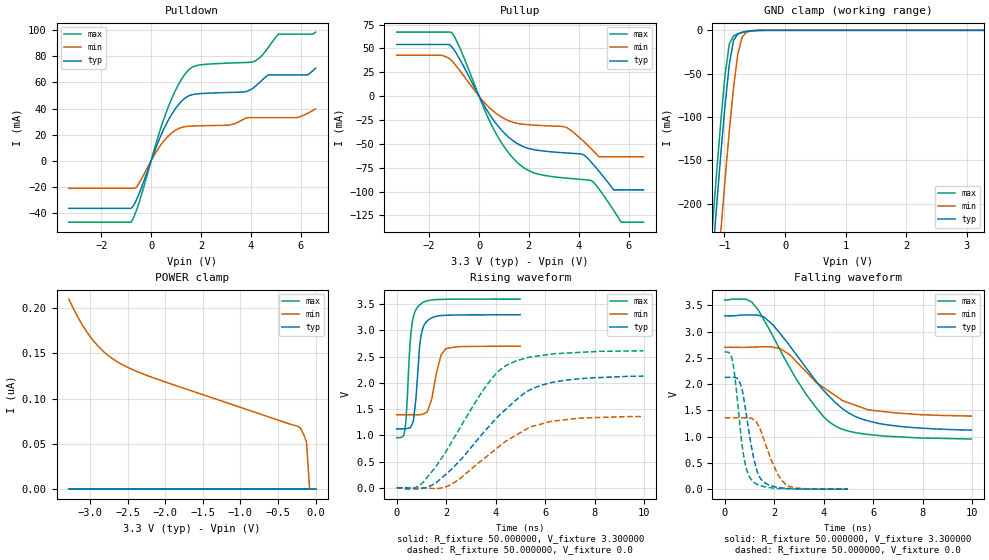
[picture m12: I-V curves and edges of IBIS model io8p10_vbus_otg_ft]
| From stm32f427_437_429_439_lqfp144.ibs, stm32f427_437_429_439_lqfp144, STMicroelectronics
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|   Model io8p10_vbus_otg_ft
[Model]  io8p10_vbus_otg_ft
Model_type I/O
Polarity   Non-Inverting
Enable   Active-Low
Vinl =   0.990000V
Vinh =   2.310000V
Vmeas =  1.650000V
Cref =   40.000000pF
Rref =   100.000000M
Vref =   0.0V
C_comp   3.304800pF   3.199300pF   3.429300pF
[Temperature Range]   25.000000   0.125000k   -40.000000
[Pullup Reference]   3.300000V   2.700000V   3.600000V
[Pulldown Reference]   0.0V   0.0V   0.0V
[POWER Clamp Reference]   3.300000V   2.700000V   3.600000V
[GND Clamp Reference]   0.0V   0.0V   0.0V
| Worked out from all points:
|   slope of the pulldown table from 0 to 0.495 V, typ, clamps not added: 20.9 ohm
|   slope of the pullup table from 0 to 0.495 V, typ, clamps not added: 22.6 ohm
|   GND clamp passes 1 mA (typ) near -0.61 V on its own axis
|   rising waveform, R_fixture 50.000000, V_fixture 3.300000: 20-80 % time 227ps typ, 354ps min, 207ps max; typ from 1.12 V to 3.3 V
|   rising waveform, R_fixture 50.000000, V_fixture 0.0: 20-80 % time 2.54ns typ, 2.33ns min, 2.1ns max; typ from 0 V to 2.13 V
|   falling waveform, R_fixture 50.000000, V_fixture 3.300000: 20-80 % time 2.29ns typ, 2.07ns min, 2.05ns max; typ from 3.3 V to 1.12 V
|   falling waveform, R_fixture 50.000000, V_fixture 0.0: 20-80 % time 481ps typ, 677ps min, 388ps max; typ from 2.13 V to 0 V
[Pulldown]
|Voltage   I(typ)   I(min)   I(max)
-3.3V     -36.41mA   -21.08mA   -47.04mA
-800mV    -36.41mA   -21.08mA   -47.04mA
-600mV    -30.48mA   -20.53mA   -38.65mA
700mV     31.4mA     19.11mA    41.71mA
1.2V      45.15mA    25.37mA    61.75mA
1.6V      50.35mA    26.5mA     71.06mA
3.1V      52.28mA    27.26mA    74.76mA
4.1V      55.7mA     33mA       75.81mA
4.7V      65.72mA    33mA       86.7mA
5.1V      65.72mA    33mA       96.91mA
6.3V      65.88mA    36.51mA    96.91mA
6.6V      70.94mA    39.72mA    98.51mA
[Pullup]
|Voltage   I(typ)   I(min)   I(max)
-3.3V     54.23mA    42.91mA    67.18mA
-1.1V     51.99mA    37.29mA    66.9mA
500mV     -22.07mA   -14mA      -30.03mA
1.5V      -49.1mA    -28.3mA    -68.56mA
2.2V      -56.05mA   -30.32mA   -80.35mA
3.5V      -59.53mA   -32.66mA   -85.92mA
4.2V      -61.44mA   -47.49mA   -87.46mA
4.5V      -69.06mA   -55.13mA   -88.4mA
4.8V      -78.23mA   -63.5mA    -96.84mA
5.4V      -98.2mA    -63.5mA    -119.6mA
5.7V      -98.2mA    -63.5mA    -132.1mA
6.6V      -98.2mA    -63.5mA    -132.1mA
[GND_clamp]
|Voltage   I(typ)   I(min)   I(max)
-3.3V     -2.321A    -2.399A    -2.294A
-1.2V     -265.6mA   -356.2mA   -227.3mA
-1.13V    -202.8mA   -293mA     -164.3mA
-1.06V    -142.3mA   -231.2mA   -104.3mA
-990mV    -86.15mA   -171.7mA   -51mA
-920mV    -39.05mA   -115.6mA   -15.71mA
-850mV    -11.4mA    -65.74mA   -6.366mA
-780mV    -4.046mA   -27.6mA    -4.153mA
-710mV    -2.285mA   -7.882mA   -2.591mA
-640mV    -1.291mA   -2.274mA   -1.367mA
-570mV    -618uA     -909.9uA   -567.3uA
3.28V     0A         0A         0A
[POWER_clamp]
|Voltage   I(typ)   I(min)   I(max)
-3.28V    0A         210.1nA    0A
-3.12V    0A         184.2nA    0A
-2.96V    0A         164.6nA    0A
-2.8V     0A         150.7nA    0A
-2.6V     0A         139nA      0A
-2.16V    0A         123.2nA    0A
-240mV    0A         69.7nA     0A
-200mV    0A         67.32nA    0A
-160mV    0A         60.72nA    0A
-120mV    0A         52.23nA    0A
-80mV     0A         0A         0A
0V        0A         0A         0A
[Ramp]
| variable   typ   min   max
dV/dt_r  1.26720/2.53271n   0.81126/2.32826n   1.56498/2.10284n
dV/dt_f  1.28280/2.27103n   0.77700/2.06011n   1.57493/2.04558n
R_load = 50.000000
[Rising Waveform]
R_fixture= 50.000000
V_fixture= 3.300000
V_fixture_min= 2.700000
V_fixture_max= 3.600000
|time   V(typ)   V(min)   V(max)
0s        1.124V     1.392V     954.4mV
300.3ps   1.126V     1.392V     1.025V
370.4ps   1.127V     1.392V     1.281V
580.6ps   1.173V     1.392V     2.99V
670.7ps   1.281V     1.391V     3.259V
850.9ps   2.211V     1.393V     3.451V
940.9ps   2.773V     1.394V     3.494V
1.111ns   3.108V     1.418V     3.548V
1.992ns   3.29V      2.655V     3.595V
4.985ns   3.3V       2.7V       3.599V
[Rising Waveform]
R_fixture= 50.000000
V_fixture= 0.0
V_fixture_min= 0.0
V_fixture_max= 0.0
|time   V(typ)   V(min)   V(max)
0s        344.1uV    194.8uV    668.7uV
460.5ps   -2.447mV   135.8uV    -26.62mV
1.041ns   -9.925mV   -1.886mV   90.32mV
1.522ns   71.01mV    -16.2mV    367.1mV
2.142ns   321.5mV    47.41mV    812.7mV
3.604ns   1.107V     586.6mV    1.936V
4.444ns   1.514V     899.1mV    2.338V
5.205ns   1.82V      1.109V     2.471V
6.166ns   1.996V     1.257V     2.544V
9.97ns    2.129V     1.359V     2.612V
[Falling Waveform]
R_fixture= 50.000000
V_fixture= 3.300000
V_fixture_min= 2.700000
V_fixture_max= 3.600000
|time   V(typ)   V(min)   V(max)
0s        3.3V       2.7V       3.599V
1.081ns   3.315V     2.702V     3.566V
1.602ns   3.273V     2.711V     3.209V
2.242ns   2.96V      2.675V     2.646V
3.303ns   2.3V       2.227V     1.798V
4.004ns   1.876V     1.932V     1.376V
4.464ns   1.654V     1.783V     1.204V
5.265ns   1.386V     1.6V       1.078V
6.226ns   1.251V     1.487V     1.021V
9.97ns    1.124V     1.392V     954.4mV
[Falling Waveform]
R_fixture= 50.000000
V_fixture= 0.0
V_fixture_min= 0.0
V_fixture_max= 0.0
|time   V(typ)   V(min)   V(max)
0s        2.129V     1.359V     2.612V
300.3ps   2.13V      1.359V     2.479V
460.5ps   2.118V     1.358V     1.944V
620.6ps   2.02V      1.358V     1.193V
850.9ps   1.492V     1.36V      432.8mV
1.111ns   736.9mV    1.343V     162.9mV
1.491ns   176.8mV    1.07V      61.14mV
2.142ns   35.36mV    283.9mV    13.96mV
2.452ns   17.46mV    97.89mV    9.223mV
4.985ns   344.1uV    194.8uV    668.7uV
